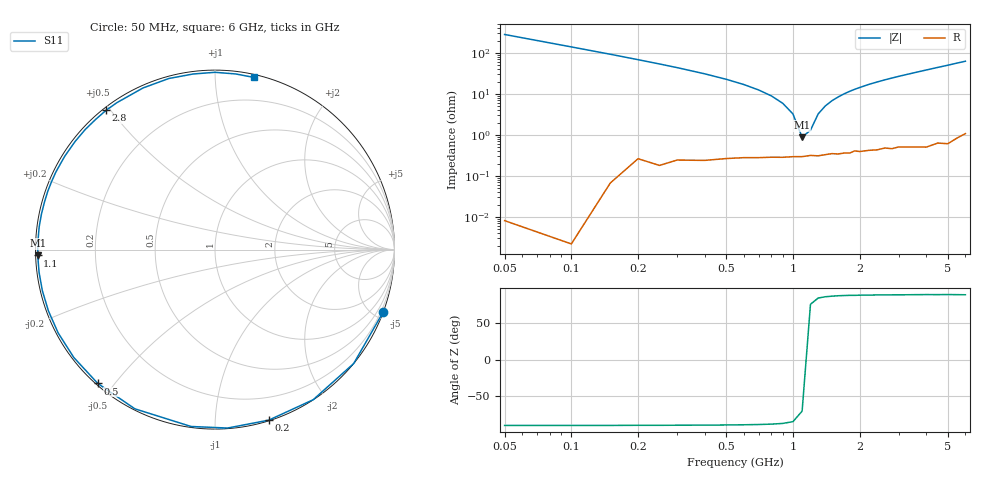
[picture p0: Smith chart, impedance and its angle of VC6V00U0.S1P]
! Infineon Technologies  Discrete & RF Semiconductors
! BBY 56-03
! Si Tuning Diode in SOD323
! VR = 6 V
! S-Parameters:  June  1999
# GHz  S  MA  R  50
!  f  S11
! GHz  MAG  ANG
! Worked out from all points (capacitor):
!   34 points, 50 MHz to 6 GHz, reference 50 ohm
!   read as one part to ground: C = 11.3 pF near 50 MHz
!   lowest |Z| = 880 mohm at 1.1 GHz (marker M1)
!   series resonance near 1.14 GHz, so ESL is about 1.7 nH
!   S11 on the Smith chart (normalised r, x): 50 MHz: 0.00, -5.61; 200 MHz: 0.01, -1.36; 500 MHz: 0.01, -0.45; 1.1 GHz: 0.01, -0.02; 2.8 GHz: 0.01, +0.49; 6 GHz: 0.02, +1.25
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0.05  1 -20.2
0.1  1 -39.4
0.15  0.9994 -56.8
0.2  0.9963 -72.5
0.25  0.9967 -86.0
0.3  0.9945 -97.7
0.4  0.9931 -116.7
0.5  0.9912 -131.2
0.6  0.99 -142.6
0.7  0.9895 -152.0
0.8  0.989 -159.8
0.9  0.9888 -166.6
1.1  0.9883 -178.1
1.3  0.9878 172.6
1.4  0.987 168.4
1.6  0.9867 160.9
1.8  0.9864 154.1
2  0.9856 148.1
2.2  0.985 142.4
2.4  0.9851 137.3
2.8  0.9852 128.0
3  0.9843 123.7
3.5  0.9858 114.0
4  0.9874 105.1
4.5  0.9859 97.1
5  0.9879 90.0
5.5  0.9853 83.2
6  0.9833 77.3
